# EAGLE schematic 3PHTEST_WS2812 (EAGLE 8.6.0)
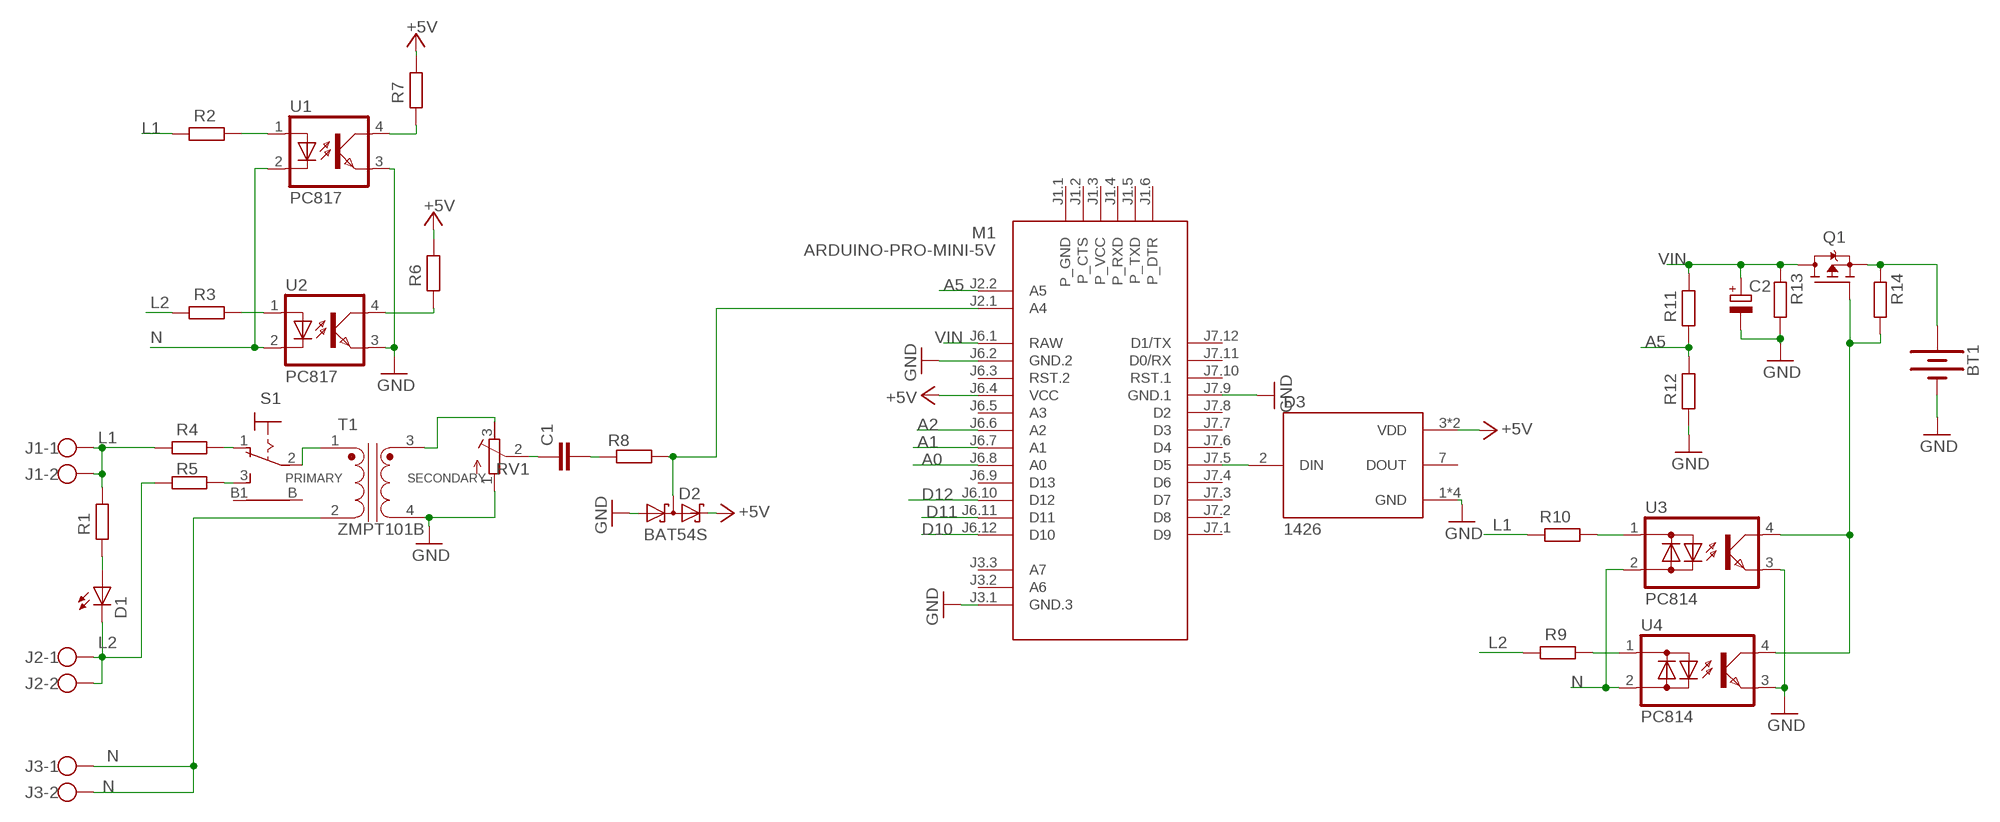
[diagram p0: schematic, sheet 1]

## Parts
BT1  BATTERY-9V  [BATTCON_9V]
C1  C-EUC1206  [C1206]
C2  CPOL-EUSMCB  [SMC_B]
D1  LED5MM  [LED5MM]
D2  BAT54S  [SOT23]
D3  1426  [LED_1426]
J1  W237-102  [W237-102]
J2  W237-102  [W237-102]
J3  W237-102  [W237-102]
M1  ARDUINO-PRO-MINI-5V  ARDUINO-PRO-MINI-3.3V  [ARDUINO-PRO-MINI]
Q1  STR2P3LLH6  [SOT23]
R1  R-EU_R2512  [R2512]
R2  R-EU_R2512  [R2512]
R3  R-EU_R2512  [R2512]
R4  R-EU_R2512  [R2512]
R5  R-EU_R2512  [R2512]
R6  R-EU_R1206  [R1206]
R7  R-EU_R1206  [R1206]
R8  R-EU_R1206  [R1206]
R9  R-EU_R2512  [R2512]
R10  R-EU_R2512  [R2512]
R11  R-EU_R1206  [R1206]
R12  R-EU_R1206  [R1206]
R13  R-EU_R1206  [R1206]
R14  R-EU_R1206  [R1206]
RV1  R-TRIMM64W  [RTRIM64W]
S1  316-917  [316-917]
T1  ZMPT101B  [XFMR_ZMPT101B]
U1  PC817  [DIL04]
U2  PC817  [DIL04]
U3  PC814  [DIL04]
U4  PC814  [DIL04]

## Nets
+5V: D2.2(C2) D3.3(VDD) D3.6(VDD) M1.J6.4(VCC) R6.1 R7.1
A0: M1.J6.8(A0)
A1: M1.J6.7(A1)
A2: M1.J6.6(A2)
A5: M1.J2.2(A5) R11.2 R12.1
D10: M1.J6.12(D10)
D11: M1.J6.11(D11)
D12: M1.J6.10(D12)
GND: BT1.- C2.- D2.1(A1) D3.1(GND) D3.4(GND) D3.5(GND) D3.8(GND) M1.J3.1(GND.3) M1.J6.2(GND.2) M1.J7.9(GND.1) R12.2 R13.2 RV1.1(A) T1.4 U1.3(EMIT) U2.3(EMIT) U3.3(E) U4.3(E)
L1: J1.1 J1.2 R1.1 R2.2 R4.2 R10.2
L2: D1.K(C) J2.1 J2.2 R3.2 R5.2 R9.2
N: J3.1 J3.2 T1.2 U1.2(C) U2.2(C) U3.2(AC2) U4.2(AC2)
N$1: BT1.+ Q1.3(S) R14.1
N$2: Q1.2(G) R14.2 U3.4(C) U4.4(C)
N$3: D2.3(C1A2) M1.J2.1(A4) R8.2
N$4: C1.1 RV1.2(S)
N$5: C1.2 R8.1
N$6: S1.2(P) T1.1
N$7: R4.1 S1.1(O)
N$8: R5.1 S1.3(S)
N$9: D3.2(DIN) M1.J7.5(D5)
N$14: R10.1 U3.1(AC1)
N$15: R9.1 U4.1(AC1)
N$18: RV1.3(E) T1.3
N$22: D1.A R1.2
N$23: R2.1 U1.1(A)
N$24: R3.1 U2.1(A)
N$25: R7.2 U1.4(COL)
N$26: R6.2 U2.4(COL)
VIN: C2.+ M1.J6.1(RAW) Q1.1(D) R11.1 R13.1
Unconnected: D3.7(DOUT) M1.J1.1(P_GND) M1.J1.2(P_CTS) M1.J1.3(P_VCC) M1.J1.4(P_RXD) M1.J1.5(P_TXD) M1.J1.6(P_DTR) M1.J3.2(A6) M1.J3.3(A7) M1.J6.3(RST.2) M1.J6.5(A3) M1.J6.9(D13) M1.J7.1(D9) M1.J7.2(D8) M1.J7.3(D7) M1.J7.4(D6) M1.J7.6(D4) M1.J7.7(D3) M1.J7.8(D2) M1.J7.10(RST.1) M1.J7.11(D0/RX) M1.J7.12(D1/TX) S1.B S1.B1

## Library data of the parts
BT1 = SparkFun-Batteries:BATTERY: Battery - Single Cell; PROD_ID: BATT-10855
C1 = rcl:C-EU: CAPACITOR, European symbol
C2 = rcl:CPOL-EU: POLARIZED CAPACITOR, European symbol
D1 = led:LED: LED
D2 = diode:BAT54S: Schottky Diodes Pin connection corrected 2011-05-04 Source: Fairchild .. BAT54.pdf
D3 = WS2812X8:1426: Check availability; AVAILABILITY: In Stock; CHECK_PRICES: https://www.snapeda.com/parts/1426/Adafruit+Industries/view-part/?ref=eda; DESCRIPTION: NeoPixel Stick - 8 x WS2812 5050 RGB LED with Integrated Drivers | Adafruit Industries 1426; MF: Adafruit; MP: 1426; PACKAGE: None; PRICE: None; SNAPEDA_LINK: https://www.snapeda.com/parts/1426/Adafruit+Industries/view-part/?ref=snap
J1-J3 = con-wago-500:W237-102: WAGO SCREW CLAMP; MPN: 237-102; OC_FARNELL: unknown; OC_NEWARK: 70K9898
M1 = diy-modules:ARDUINO-PRO-MINI-*: Arduino Pro Mini and compatible devices More details available here: https://www.arduino.cc/en/Main/ArduinoBoardProMini Click here to find device on ebay.com
Q1 = transistor-fet:STR2P3LLH6
R1-R14 = rcl:R-EU_: RESISTOR, European symbol
RV1 = rcl:R-TRIMM: Trimm resistor
S1 = switch:316-917: TOGGLE SWITCH Mors, distributor RS Components
T1 = ZMPT101B:ZMPT101B: Check availability; AVAILABILITY: Not in stock; CHECK_PRICES: https://www.snapeda.com/parts/ZMPT101B/Qingxian+Zeming+Langxi+Electronic/view-part/?ref=eda; DESCRIPTION: Current-type Voltage Transformer; MF: Qingxian Zeming Langxi Electronic; MP: ZMPT101B; PACKAGE: None; PRICE: None; SNAPEDA_LINK: https://www.snapeda.com/parts/ZMPT101B/Qingxian+Zeming+Langxi+Electronic/view-part/?ref=snap
U1 U2 = optocoupler:PC817: SHARP OPTO COUPLER; MPN: PC817X4J000F; OC_FARNELL: 9707727; OC_NEWARK: 97K7059
U3 U4 = optocoupler:PC814: SHARP OPTO COUPLER; OC_FARNELL: 9707662; OC_NEWARK: unknown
